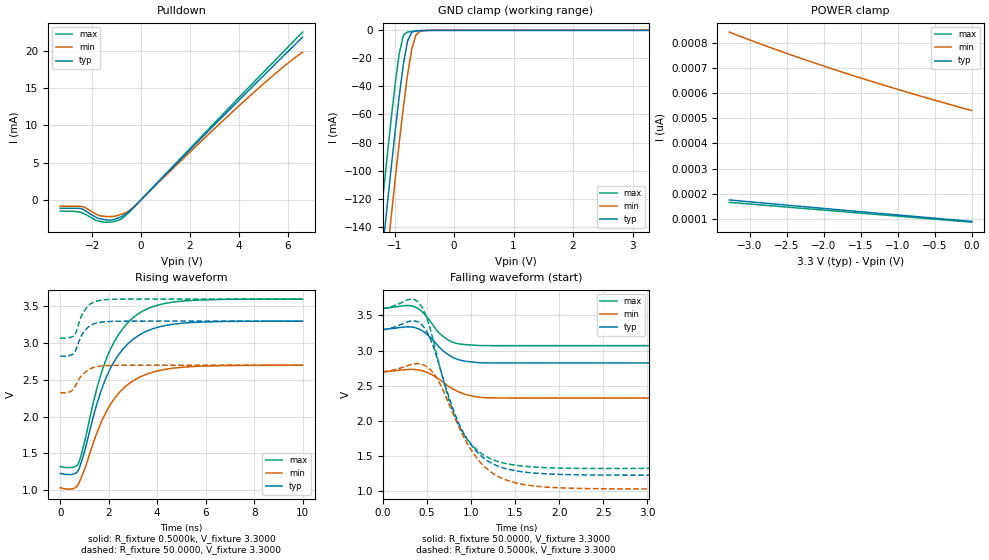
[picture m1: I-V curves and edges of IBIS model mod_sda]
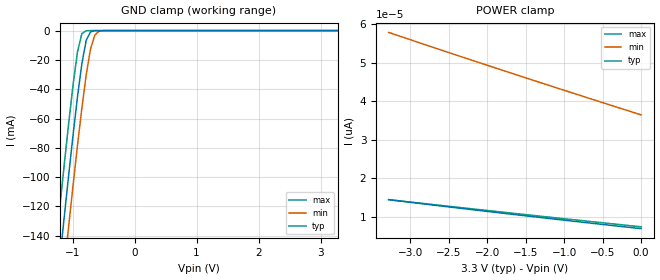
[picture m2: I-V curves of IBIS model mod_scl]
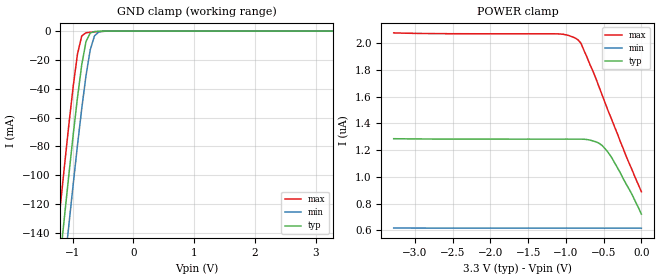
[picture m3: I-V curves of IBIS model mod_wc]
| IBIS (I/O, Buffer, Information, Specification) Model, officially
| electronic behavioral standard for Buffer structures of digital pins.
[IBIS ver]  4.0
[File name] m24c16_fc2_tssop8.ibs
[File Rev]  1.0
[Date]   24 Sept 2014
[Source]   CAD & Design Services (Catania) - STMicroelectronics
[Notes]
   (Note1)  This IBIS model includes the TSSOP8 package data
   (Note2)  This IBIS model has some Notes about the non-monotonicity
   of the I-V curves, but they are not indicative of problems
   inside the model;
[Copyright] (c) 2014 STMicroelectronics
|   Component M24C16
[Component] M24C16
[Manufacturer] STMicroelectronics
[Package]
| variable   typ   min   max
R_pkg   0.0   0.0   0.0
L_pkg   0.0H   0.0H   0.0H
C_pkg   0.0F   0.0F   0.0F
[Pin]  signal_name   model_name   R_pin   L_pin   C_pin
1   1NC   NC   NA   NA   NA
2   2NC   NC   NA   NA   NA
3   3NC   NC   NA   NA   NA
4   VSS   GND   NA   NA   NA
5   SDA   mod_sda   NA   NA   NA
6   SCL   mod_scl   NA   NA   NA
7   WCN   mod_wc   NA   NA   NA
8   VCC   POWER   NA   NA   NA
[Package Model]  182696_TSSOP8
[Define Package Model]  182696_TSSOP8
[Manufacturer]  STMicroelectronics
[OEM]  STMicroelectronics
[Description]  8 pin TSSOP package
[Number Of Pins]  8
[Pin Numbers]
|Pin Num   Terminal Name
1   | net1
2   | net2
3   | net3
4   | net4_GND
5   | net5
6   | net6
7   | net7
8   | net8_VDD
[Model Data]
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[End Model Data]
[End Package Model]
| Models and submodels in the file (3): mod_sda (I/O_open_drain), mod_scl (Input), mod_wc (Input)
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|   Model mod_sda
[Model]   mod_sda
Model_type I/O_open_drain
Vinl   =   1.000V
Vinh   =   2.300V
Vmeas  =   1.650V
Cref   =   10pF
Rref   =   1k
Vref   =   3.3000V
C_comp   1.846pF   1.683pF   1.932pF
[Temperature Range]   25.0000   85.0000   -40.0000
[Voltage Range]   3.3000V   2.7000V   3.6000V
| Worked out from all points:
|   slope of the pulldown table from 0 to 0.495 V, typ, clamps not added: 296 ohm
|   GND clamp passes 1 mA (typ) near -0.69 V on its own axis
|   rising waveform, R_fixture 0.5000k, V_fixture 3.3000: 20-80 % time 1.41ns typ, 1.46ns min, 1.38ns max; typ from 1.23 V to 3.3 V
|   rising waveform, R_fixture 50.0000, V_fixture 3.3000: 20-80 % time 461ps typ, 514ps min, 433ps max; typ from 2.83 V to 3.3 V
|   falling waveform, R_fixture 50.0000, V_fixture 3.3000: 20-80 % time 247ps typ, 285ps min, 221ps max; typ from 3.3 V to 2.83 V
|   falling waveform, R_fixture 0.5000k, V_fixture 3.3000: 20-80 % time 396ps typ, 432ps min, 364ps max; typ from 3.3 V to 1.23 V
[Pulldown]
|Voltage   I(typ)   I(min)   I(max)
-3.3V     -1.144mA   -880uA     -1.546mA
-2.4V     -1.247mA   -920uA     -1.771mA
-1.8V     -2.432mA   -2.016mA   -2.814mA
-1.5V     -2.674mA   -2.237mA   -3.003mA
-1.2V     -2.725mA   -2.257mA   -2.994mA
-900mV    -2.41mA    -2.064mA   -2.727mA
-700mV    -2.089mA   -1.845mA   -2.343mA
-300mV    -1.015mA   -975.8uA   -1.037mA
2.3V      7.74mA     7.374mA    7.927mA
4.4V      14.72mA    13.83mA    15.11mA
5.7V      18.97mA    17.57mA    19.53mA
6.6V      21.88mA    19.88mA    22.58mA
[GND_clamp]
|Voltage   I(typ)   I(min)   I(max)
-3.3V     -1.071A    -1.104A    -1.039A
-1.27V    -185.2mA   -220.4mA   -149.9mA
-1.2V     -156.1mA   -191.3mA   -120.7mA
-1.13V    -127.3mA   -162.4mA   -92.06mA
-1.06V    -99.14mA   -134mA     -64.31mA
-920mV    -46.16mA   -79.3mA    -15.94mA
-850mV    -23.46mA   -53.85mA   -3.377mA
-780mV    -7.326mA   -30.95mA   -1.138mA
-710mV    -1.308mA   -12.96mA   -800.3uA
-640mV    -333.4uA   -3.282mA   -566uA
-570mV    -139.5uA   -643.1uA   -346.9uA
3.28V     89.02pA    579.4pA    78.63pA
[POWER_clamp]
|Voltage   I(typ)   I(min)   I(max)
-3.28V    175.1pA    844.1pA    165.4pA
-2.84V    163.3pA    794.8pA    154.7pA
-2.56V    155.8pA    765pA      148pA
-1.8V     135.8pA    689.1pA    129.6pA
-920mV    113pA      608.7pA    108.4pA
0V        89.53pA    531.4pA    86.32pA
[Ramp]
| variable   typ   min   max
dV/dt_r   0.2848/0.5188n   0.2237/0.5810n   0.3172/0.4858n
dV/dt_f   0.2848/0.2721n   0.2237/0.3163n   0.3172/0.2423n
R_load = 50.0000
[Rising Waveform]
R_fixture= 0.5000k
V_fixture= 3.3000
V_fixture_min= 2.7000
V_fixture_max= 3.6000
|time   V(typ)   V(min)   V(max)
0s        1.228V     1.032V     1.321V
500ps     1.216V     1.019V     1.311V
760ps     1.281V     1.092V     1.373V
1.5ns     2.158V     1.768V     2.37V
1.92ns    2.55V      2.079V     2.801V
2.47ns    2.871V     2.34V      3.147V
3.2ns     3.098V     2.524V     3.395V
4ns       3.214V     2.621V     3.515V
5.18ns    3.275V     2.676V     3.577V
10ns      3.3V       2.7V       3.6V
[Rising Waveform]
R_fixture= 50.0000
V_fixture= 3.3000
V_fixture_min= 2.7000
V_fixture_max= 3.6000
|time   V(typ)   V(min)   V(max)
0s        2.825V     2.327V     3.071V
380ps     2.832V     2.336V     3.076V
560ps     2.863V     2.384V     3.099V
660ps     2.924V     2.441V     3.156V
880ps     3.106V     2.56V      3.377V
1.06ns    3.185V     2.612V     3.471V
1.3ns     3.25V      2.661V     3.545V
1.64ns    3.283V     2.687V     3.582V
2.66ns    3.299V     2.699V     3.599V
10ns      3.3V       2.7V       3.6V
[Falling Waveform]
R_fixture= 50.0000
V_fixture= 3.3000
V_fixture_min= 2.7000
V_fixture_max= 3.6000
|time   V(typ)   V(min)   V(max)
0s        3.3V       2.7V       3.6V
260ps     3.337V     2.73V      3.641V
350ps     3.333V     2.733V     3.629V
430ps     3.296V     2.72V      3.571V
530ps     3.201V     2.676V     3.433V
630ps     3.066V     2.603V     3.266V
750ps     2.938V     2.491V     3.147V
890ps     2.862V     2.4V       3.092V
1.09ns    2.83V      2.339V     3.074V
10ns      2.825V     2.327V     3.071V
[Falling Waveform]
R_fixture= 0.5000k
V_fixture= 3.3000
V_fixture_min= 2.7000
V_fixture_max= 3.6000
|time   V(typ)   V(min)   V(max)
0s        3.3V       2.7V       3.6V
410ps     3.403V     2.814V     3.681V
510ps     3.246V     2.763V     3.427V
610ps     2.919V     2.616V     2.958V
770ps     2.269V     2.184V     2.23V
890ps     1.893V     1.845V     1.874V
1.13ns    1.489V     1.38V      1.529V
1.41ns    1.318V     1.157V     1.392V
2.41ns    1.233V     1.039V     1.326V
10ns      1.228V     1.032V     1.321V
|   Model mod_scl
[Model]   mod_scl
Model_type Input
Enable   Active-High
Vinl   =   1.000V
Vinh   =   2.300V
C_comp   1.763pF   1.683pF   1.932pF
[Temperature Range]  25.0000   85.0000   -40.0000
[Voltage Range]   3.3000V   2.7000V   3.6000V
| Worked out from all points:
|   GND clamp passes 1 mA (typ) near -0.71 V on its own axis
[GND_clamp]
|Voltage   I(typ)   I(min)   I(max)
-3.3V     -1.062A    -1.095A    -1.029A
-1.27V    -183mA     -218.2mA   -147.1mA
-1.2V     -154mA     -189.3mA   -118.2mA
-1.13V    -125.5mA   -160.7mA   -89.81mA
-1.06V    -97.6mA    -132.5mA   -62.31mA
-920mV    -45.09mA   -78.25mA   -14.43mA
-850mV    -22.62mA   -53.01mA   -2.105mA
-780mV    -6.701mA   -30.31mA   -106.4uA
-710mV    -882.5uA   -12.5mA    -4.426uA
-640mV    -77.69uA   -2.963mA   -182.3nA
-570mV    -6.449uA   -439.6uA   -7.506nA
3.28V     6.812pA    40.1pA     6.665pA
[POWER_clamp]
|Voltage   I(typ)   I(min)   I(max)
-3.28V    14.38pA    57.84pA    14.39pA
-2.52V    12.55pA    52.74pA    12.71pA
-1.72V    10.69pA    47.47pA    10.97pA
0V        6.856pA    36.42pA    7.331pA
|   Model mod_wc
[Model]   mod_wc
Model_type Input
Enable   Active-High
Vinl   =   1.000V
Vinh   =   2.300V
C_comp   1.763pF   1.683pF   1.932pF
[Temperature Range]  25.0000   85.0000   -40.0000
[Voltage Range]   3.3000V   2.7000V   3.6000V
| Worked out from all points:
|   GND clamp passes 1 mA (typ) near -0.69 V on its own axis
[GND_clamp]
|Voltage   I(typ)   I(min)   I(max)
-3.3V     -1.071A    -1.104A    -1.039A
-1.27V    -185.2mA   -220.4mA   -149.9mA
-1.2V     -156.1mA   -191.3mA   -120.7mA
-1.13V    -127.3mA   -162.4mA   -92.06mA
-1.06V    -99.14mA   -134mA     -64.31mA
-920mV    -46.16mA   -79.3mA    -15.94mA
-850mV    -23.46mA   -53.85mA   -3.377mA
-780mV    -7.326mA   -30.95mA   -1.138mA
-710mV    -1.308mA   -12.96mA   -800.3uA
-640mV    -333.4uA   -3.282mA   -566uA
-570mV    -139.5uA   -643.1uA   -346.9uA
3.28V     89.02pA    579.4pA    78.63pA
[POWER_clamp]
|Voltage   I(typ)   I(min)   I(max)
-3.28V    1.285uA    617.9nA    2.075uA
-1.12V    1.282uA    616.7nA    2.068uA
-960mV    1.282uA    616.7nA    2.056uA
-840mV    1.282uA    616.7nA    2.024uA
-800mV    1.282uA    616.7nA    1.998uA
-600mV    1.261uA    616.7nA    1.731uA
-520mV    1.234uA    616.6nA    1.612uA
-480mV    1.21uA     616.6nA    1.552uA
-400mV    1.15uA     616.6nA    1.438uA
-280mV    1.031uA    616.6nA    1.266uA
-120mV    864nA      616.6nA    1.048uA
0V        721.6nA    616.6nA    888.6nA
